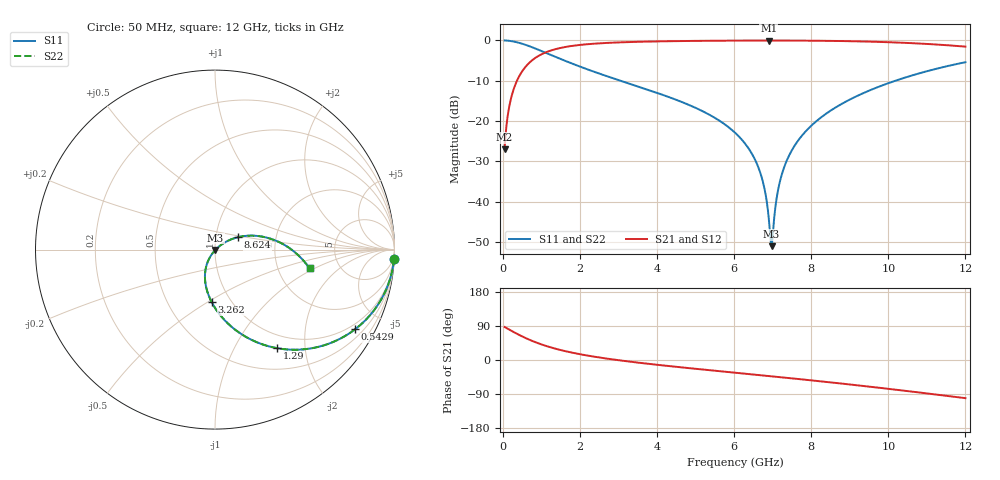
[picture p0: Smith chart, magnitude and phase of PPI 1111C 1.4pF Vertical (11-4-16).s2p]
# GHz S MA R 50
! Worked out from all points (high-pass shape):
!   1601 points, 50 MHz to 12 GHz, reference 50 ohm
!   highest |S21| = -0.03 dB at 6.899 GHz (marker M1); lowest = -27.0 dB at 50 MHz (marker M2)
!   |S21| within 3 dB of the highest: 1.101 GHz to end of sweep
!   lowest |S11| = -51.0 dB at 6.974 GHz (marker M3), VSWR 1.01, Z = 50.2 - j0.178 ohm
!   |S11| at or under -10 dB: 3.057 GHz to 10.18 GHz (7.126 GHz wide, 108 % of centre)
!   |S22| runs from -51.0 to 0.0 dB; largest |S21 - S12| = 0
!   S11 on the Smith chart (normalised r, x): 50 MHz: 1, -39; 542.9 MHz: 0.79, -3.63; 1.29 GHz: 0.79, -1.50; 3.262 GHz: 0.81, -0.52; 8.624 GHz: 1.28, +0.18; 12 GHz: 3.03, -0.89
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0.05  0.999 -2.9  0.04491 87.1  0.04491 87.1  0.999 -2.9
0.1545625  0.9905 -8.9  0.1377 81.1  0.1377 81.1  0.9905 -8.9
0.2367188  0.978 -13.6  0.2082 76.4  0.2082 76.4  0.978 -13.6
0.5429375  0.8981 -29.6  0.4392 60.4  0.4392 60.4  0.8981 -29.6
1.289813  0.6484 -57.9  0.7603 32.0  0.7603 32.0  0.6484 -57.9
2.044156  0.466 -75.3  0.8834 14.5  0.8834 14.5  0.466 -75.3
3.261563  0.2936 -93.6  0.9541 -3.9  0.9541 -3.9  0.2936 -93.6
4.038312  0.2207 -102.5  0.9732 -13.0  0.9732 -13.0  0.2207 -102.5
5.24825  0.128 -114.7  0.9893 -25.7  0.9893 -25.7  0.128 -114.7
6.025  0.07182 -121.6  0.9946 -33.5  0.9946 -33.5  0.07182 -121.6
6.6225  0.0273 -123.9  0.9966 -39.5  0.9966 -39.5  0.0273 -123.9
6.786812  0.01475 -120.5  0.9968 -41.1  0.9968 -41.1  0.01475 -120.5
6.898844  0.006357 -106.4  0.9968 -42.3  0.9968 -42.3  0.006357 -106.4
6.973531  0.002813 -39.2  0.9968 -43.0  0.9968 -43.0  0.002813 -39.2
7.010875  0.004239 4.9  0.9968 -43.4  0.9968 -43.4  0.004239 4.9
7.145313  0.01427 33.6  0.9966 -44.8  0.9966 -44.8  0.01427 33.6
7.309625  0.02759 37.4  0.9963 -46.5  0.9963 -46.5  0.02759 37.4
7.600906  0.0521 37.2  0.9952 -49.5  0.9952 -49.5  0.0521 37.2
8.019156  0.08907 34.1  0.9924 -53.8  0.9924 -53.8  0.08907 34.1
8.624125  0.1465 28.3  0.9852 -60.4  0.9852 -60.4  0.1465 28.3
10.01331  0.2964 13.0  0.9503 -76.2  0.9503 -76.2  0.2964 13.0
12  0.5368 -11.2  0.8378 -100.7  0.8378 -100.7  0.5368 -11.2
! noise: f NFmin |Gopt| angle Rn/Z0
0.05  0.0008132  0.9581  2.12  0.004371
1.372  0.004094  0.7029  11.85  0.002674
2.701  0.006406  0.6407  19.67  0.003275
4.031  0.008494  0.611  27.35  0.003837
5.36  0.01053  0.5986  34.68  0.004426
6.682  0.0126  0.5981  41.56  0.005089
8.012  0.01482  0.6068  48.04  0.005885
9.341  0.01725  0.6229  54.11  0.006874
10.67  0.01999  0.6451  59.81  0.008141
12  0.02316  0.6722  65.2  0.009806
